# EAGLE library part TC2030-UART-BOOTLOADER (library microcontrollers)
TAG-CONNECT ICSP Connector Manufacturer: Tag-Connect Cable for easy In-Circuit Serial Programming. Designed for Microchip ICD2, suitable for many others. Two variants - one "with legs" (for hands-free fit on PCB) and another "without legs" for quick programming. PADDescription 1MCLR/Vpp 2Vdd 3GND 4PGD (ISPDAT) 5PGC (ISPCLK) 6nc (used for LVP) ©2009 ROFA.cz - modified and updated by Robert Darlington &#8249;rdarlington@gmail.com&#8250;
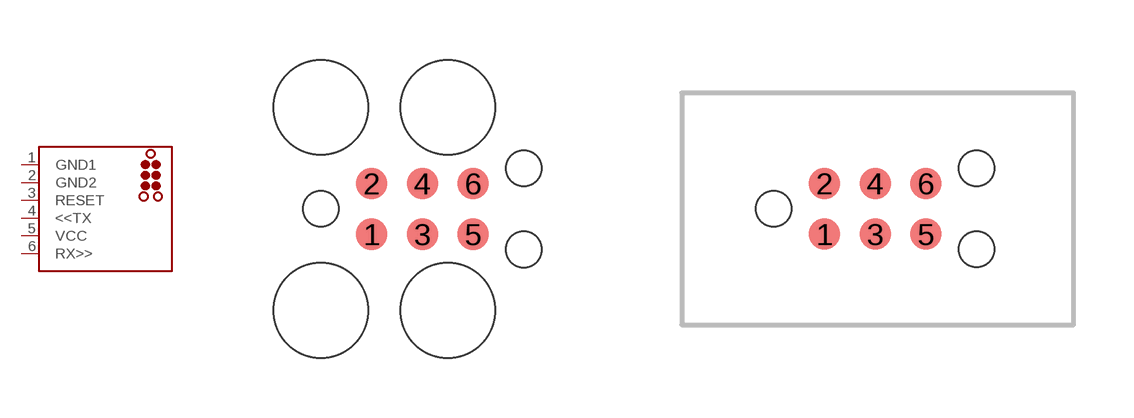
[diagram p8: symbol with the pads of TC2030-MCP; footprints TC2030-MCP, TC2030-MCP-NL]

Designator prefix J

## TC2030-UART-BOOTLOADER-MCP  [TC2030-MCP]
1  GND1  pwr
2  GND2  pwr
3  RESET  pwr
4  <<TX  pwr
5  VCC  in
6  RX>>

## TC2030-UART-BOOTLOADER-MCP-NL  [TC2030-MCP-NL]
Pads as for TC2030-MCP

## Footprint TC2030-MCP (pad centres in mm)
TAG-CONNECT ICSP Connector - Legged version Manufacturer: Tag-Connect Cable for easy In-Circuit Serial Programming. Designed for Microchip ICD2, suitable for many others. NOTE: Eagle's default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
smd 0.787 x 0.787: 1 1.27,-0.635; 2 1.27,0.635; 3 2.54,-0.635; 4 2.54,0.635; 5 3.81,-0.635; 6 3.81,0.635
hole 0.889 at 0,0
hole 0.889 at 5.08,-1.016
hole 0.889 at 5.08,1.016
hole 2.375 at 0,2.54
hole 2.375 at 0,-2.54
hole 2.375 at 3.175,-2.54
hole 2.375 at 3.175,2.54

## Footprint TC2030-MCP-NL (pad centres in mm)
TAG-CONNECT ICSP Connector Manufacturer: Tag-Connect Cable for easy In-Circuit Serial Programming. Designed for Microchip ICD2, suitable for many others. PADDescription 1MCLR/Vpp 2Vdd 3GND 4PGD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
smd 0.787 x 0.787: 1 1.27,-0.635; 2 1.27,0.635; 3 2.54,-0.635; 4 2.54,0.635; 5 3.81,-0.635; 6 3.81,0.635
hole 0.889 at 0,0
hole 0.889 at 5.08,-1.016
hole 0.889 at 5.08,1.016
